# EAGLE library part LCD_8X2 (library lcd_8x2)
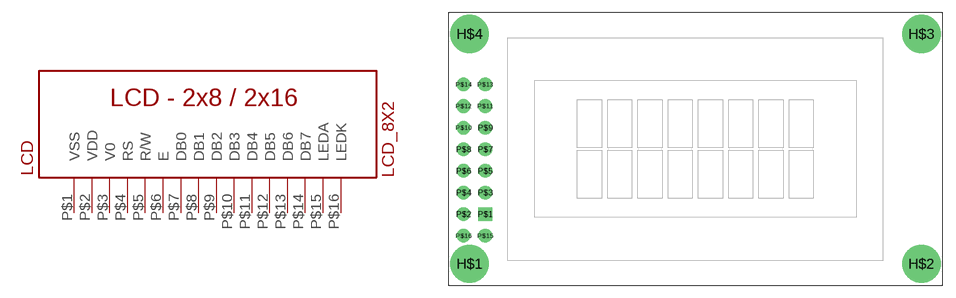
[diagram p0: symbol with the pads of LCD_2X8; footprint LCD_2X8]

Designator prefix LCD

## LCD_8X2  [LCD_2X8]
P$1  VSS  pwr
P$2  VDD  pwr
P$3  V0
P$4  RS
P$5  R/W
P$6  E
P$7  DB0
P$8  DB1
P$9  DB2
P$10  DB3
P$11  DB4
P$12  DB5
P$13  DB6
P$14  DB7
P$15  LEDA  pwr
P$16  LEDK  pwr

## Footprint LCD_2X8 (pad centres in mm)
drill 3 pad 4.5: H$1 2.5,2.5; H$2 55.5,2.5; H$3 55.5,29.5; H$4 2.5,29.5
drill 0.9 pad 1.6 square: P$1 4.34,8.34
drill 0.9 pad 1.6: P$2 1.8,8.34; P$3 4.34,10.88; P$4 1.8,10.88; P$5 4.34,13.42; P$6 1.8,13.42; P$7 4.34,15.96; P$8 1.8,15.96; P$9 4.34,18.5; P$10 1.8,18.5; P$11 4.34,21.04; P$12 1.8,21.04; P$13 4.34,23.58; P$14 1.8,23.58; P$15 4.34,5.8; P$16 1.8,5.8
